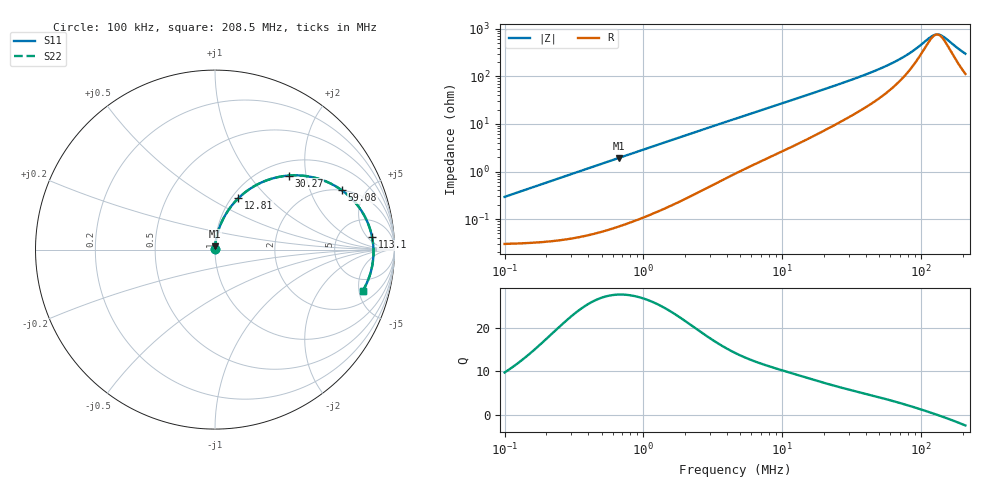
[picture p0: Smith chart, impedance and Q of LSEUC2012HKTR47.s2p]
! LSEUC2012HKTR47  S-PARAMETER MODEL  ( General Type )
! Model Generated by TAIYO YUDEN Corporation (http://www.ty-top.com)
! Version 1.0
! TAIYO YUDEN Control No. 211126
! Copyright(c) 2021 TAIYO YUDEN CO.,LTD. All Rights Reserved.
! Product Description (link to TY-COMPAS)
! https://ds.yuden.co.jp/TYCOMPAS/or/detail?pn=LSEUC2012HKTR47M&u=M
! Products Name : Inductors
! Characteristics :
!  Inductance : 0.47 uH , SRF(min) : -Hz , DC Resistance(max) : 0.033 Ohm
!  Rated Current : Saturation :4500 mA , Temp Rise : 3800 mA (40 degC)
!  Case Size : 2.0 x 1.2 / 0.079 x 0.047 [mm/inch] , Thickness : 0.8 / 0.031 [mm/inch]
!  (Conditions: Temperature = 25 degC , DC Bias Current/Voltage = 0A / 0V)
! External Node Assignments :
!  1  o---GGG---o  2
! GND o---------o GND
! Frequency Range : 0.1MHz  -  208.503118MHz  [ 402 STEP ]
# MHz S RI R 50
! Freq[MHz].  S11 Real  S11 Imag  S21 Real  S21 Imag  S12 Real  S12 Imag  S22 Real  S22 Imag
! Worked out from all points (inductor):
!   401 points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, 100 kHz to 208.5 MHz, reference 50 ohm
!   read as one part in series: L = 465 nH near 103.9 kHz
!   highest Q = 27.5 at 662.9 kHz (marker M1), where L = 461 nH
!   self-resonance near 130.1 MHz
!   S11 on the Smith chart (normalised r, x): 100 kHz: 1.00, +0.01; 12.81 MHz: 1.07, +0.68; 30.27 MHz: 1.28, +1.59; 59.08 MHz: 2.01, +3.39; 113.1 MHz: 11, +7; 208.5 MHz: 3.24, -5.51
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0.1  0.00031 0.00292  0.9997 -0.00292  0.9997 -0.00292  0.00031 0.00292
0.359709  0.000538 0.0105  0.9995 -0.0105  0.9995 -0.0105  0.000538 0.0105
0.662949  0.00106 0.0192  0.9989 -0.0192  0.9989 -0.0192  0.00106 0.0192
1.293906  0.00285 0.037  0.9972 -0.037  0.9972 -0.037  0.00285 0.037
2.574085  0.00906 0.0721  0.9909 -0.0721  0.9909 -0.0721  0.00906 0.0721
4.654297  0.0252 0.1251  0.9748 -0.1251  0.9748 -0.1251  0.0252 0.1251
8.256339  0.0651 0.2054  0.9349 -0.2054  0.9349 -0.2054  0.0651 0.2054
12.81258  0.1306 0.2866  0.8694 -0.2866  0.8694 -0.2866  0.1306 0.2866
16.42508  0.1891 0.3348  0.8109 -0.3348  0.8109 -0.3348  0.1891 0.3348
21.87632  0.2799 0.3828  0.7201 -0.3828  0.7201 -0.3828  0.2799 0.3828
30.27169  0.4104 0.4126  0.5896 -0.4126  0.5896 -0.4126  0.4104 0.4126
42.69694  0.5664 0.3977  0.4336 -0.3977  0.4336 -0.3977  0.5664 0.3977
59.08252  0.7073 0.3303  0.2927 -0.3303  0.2927 -0.3303  0.7073 0.3303
70.16799  0.7704 0.2745  0.2296 -0.2745  0.2296 -0.2745  0.7704 0.2745
81.75631  0.8164 0.2152  0.1836 -0.2152  0.1836 -0.2152  0.8164 0.2152
93.45569  0.8475 0.1575  0.1525 -0.1575  0.1525 -0.1575  0.8475 0.1575
113.1315  0.8754 0.0682  0.1246 -0.0682  0.1246 -0.0682  0.8754 0.0682
124.4722  0.8818 0.0216  0.1182 -0.0216  0.1182 -0.0216  0.8818 0.0216
136.9498  0.8829 -0.0256  0.1171 0.0256  0.1171 0.0256  0.8829 -0.0256
147.8266  0.88 -0.0634  0.12 0.0634  0.12 0.0634  0.88 -0.0634
185.9199  0.8507 -0.1751  0.1493 0.1751  0.1493 0.1751  0.8507 -0.1751
208.5031  0.8244 -0.228  0.1756 0.228  0.1756 0.228  0.8244 -0.228
